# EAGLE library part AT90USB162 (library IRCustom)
MICROCONTROLLER 8 Kbytes FLASH 1 kbytes SRAM 512 bytes EEPROM USART 6-channel 10 bit ADC 2-channel 8 bit ADC
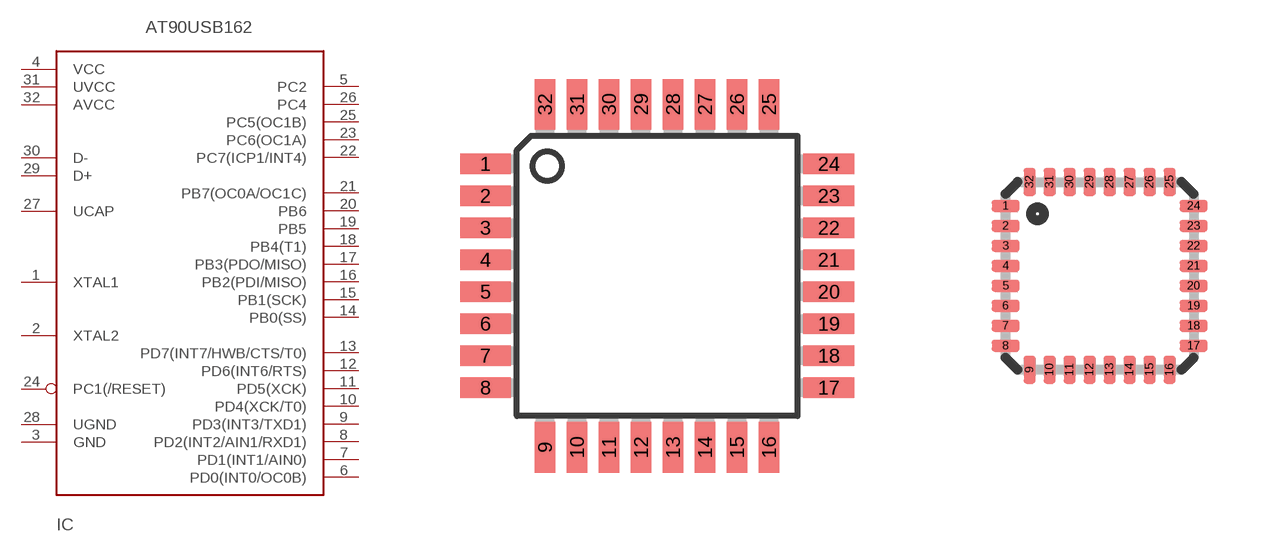
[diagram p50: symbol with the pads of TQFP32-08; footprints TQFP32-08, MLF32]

Designator prefix IC

## AT90USB162A  [TQFP32-08]
1  XTAL1
2  XTAL2
3  GND
4  VCC
5  PC2
6  PD0(INT0/OC0B)
7  PD1(INT1/AIN0)
8  PD2(INT2/AIN1/RXD1)
9  PD3(INT3/TXD1)
10  PD4(XCK/T0)
11  PD5(XCK)
12  PD6(INT6/RTS)
13  PD7(INT7/HWB/CTS/T0)
14  PB0(SS)
15  PB1(SCK)
16  PB2(PDI/MISO)
17  PB3(PDO/MISO)
18  PB4(T1)
19  PB5
20  PB6
21  PB7(OC0A/OC1C)
22  PC7(ICP1/INT4)
23  PC6(OC1A)
24  PC1(/RESET)
25  PC5(OC1B)
26  PC4
27  UCAP
28  UGND
29  D+
30  D-
31  UVCC
32  AVCC

## AT90USB162QFN  [MLF32]
Pads as for TQFP32-08

## Footprint TQFP32-08 (pad centres in mm)
Thin Plasic Quad Flat Package Grid 0.8 mm
smd 1.27 x 0.508: 1 -4.293,2.8; 2 -4.293,2; 3 -4.293,1.2; 4 -4.293,0.4; 5 -4.293,-0.4; 6 -4.293,-1.2; 7 -4.293,-2; 8 -4.293,-2.8; 17 4.293,-2.8; 18 4.293,-2; 19 4.293,-1.2; 20 4.293,-0.4; 21 4.293,0.4; 22 4.293,1.2; 23 4.293,2; 24 4.293,2.8
smd 0.508 x 1.27: 9 -2.8,-4.293; 10 -2,-4.293; 11 -1.2,-4.293; 12 -0.4,-4.293; 13 0.4,-4.293; 14 1.2,-4.293; 15 2,-4.293; 16 2.8,-4.293; 25 2.8,4.293; 26 2,4.293; 27 1.2,4.293; 28 0.4,4.293; 29 -0.4,4.293; 30 -1.2,4.293; 31 -2,4.293; 32 -2.8,4.293

## Footprint MLF32 (pad centres in mm)
32M1-A Micro Lead Frame package (MLF) Source: http://www.atmel.com .. doc1477.pdf
smd 0.7 x 0.3: 1 -2.35,1.75; 2 -2.35,1.25; 3 -2.35,0.75; 4 -2.35,0.25; 5 -2.35,-0.25; 6 -2.35,-0.75; 7 -2.35,-1.25; 8 -2.35,-1.75; 17 2.35,-1.75; 18 2.35,-1.25; 19 2.35,-0.75; 20 2.35,-0.25; 21 2.35,0.25; 22 2.35,0.75; 23 2.35,1.25; 24 2.35,1.75
smd 0.3 x 0.7: 9 -1.75,-2.35; 10 -1.25,-2.35; 11 -0.75,-2.35; 12 -0.25,-2.35; 13 0.25,-2.35; 14 0.75,-2.35; 15 1.25,-2.35; 16 1.75,-2.35; 25 1.75,2.35; 26 1.25,2.35; 27 0.75,2.35; 28 0.25,2.35; 29 -0.25,2.35; 30 -0.75,2.35; 31 -1.25,2.35; 32 -1.75,2.35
